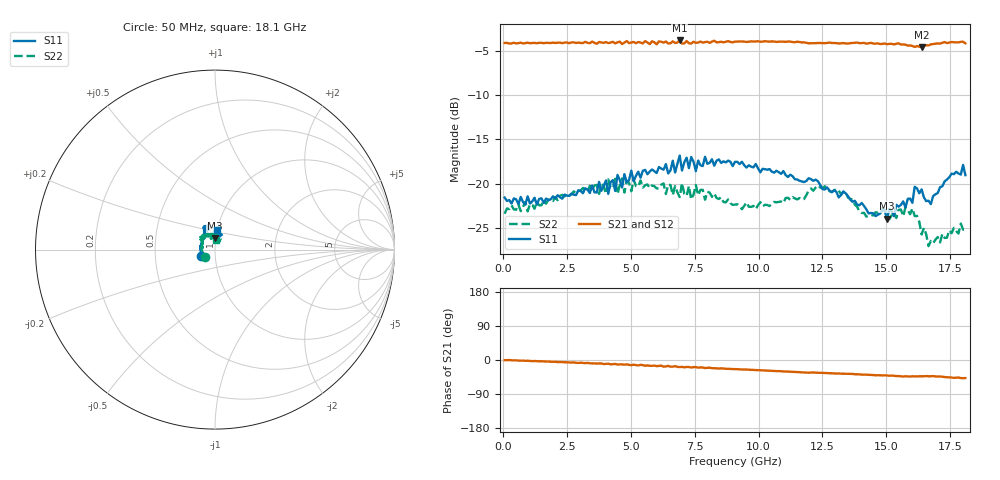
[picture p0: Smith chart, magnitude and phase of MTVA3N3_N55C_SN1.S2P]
! Network Analyzer HP8720D.06.14 Serial No. US36140669
! 27 Jun 2005  08:34:29
! Frequency  S11  S21  S12  S22
# HZ  S  DB R 50
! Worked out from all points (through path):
!   201 points, 50 MHz to 18.1 GHz, reference 50 ohm
!   highest |S21| = -3.81 dB at 6.909 GHz (marker M1); lowest = -4.6 dB at 16.39 GHz (marker M2)
!   group delay of S21, straight-line fit = 7.54 ps
!   lowest |S11| = -24.0 dB at 15.03 GHz (marker M3), VSWR 1.14, Z = 49.6 + j6.31 ohm
!   |S11| at or under -10 dB: start of sweep to end of sweep
!   |S22| runs from -27.1 to -19.4 dB; largest |S21 - S12| = 0.02
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5e7  -21.58 -155.5  -4.09 -0.5  -4.12 -0.1  -23.41 -142.0
3.1185e9  -21.09 137.7  -4.11 -7.8  -4.11 -8.0  -20.50 144.8
6.09675e9  -18.13 115.8  -3.91 -15.7  -3.90 -15.5  -20.54 123.5
6.45775e9  -18.86 118.1  -4.15 -15.4  -4.18 -16.4  -20.11 118.0
6.63825e9  -17.42 115.3  -3.90 -17.6  -4.03 -16.9  -21.31 117.9
6.7285e9  -18.75 117.8  -4.09 -16.2  -4.17 -17.4  -20.28 115.8
6.909e9  -16.83 114.8  -3.81 -18.5  -4.00 -17.9  -21.53 112.7
6.99925e9  -18.53 113.1  -4.15 -18.1  -4.11 -19.4  -19.95 113.7
7.36025e9  -16.99 104.8  -4.16 -19.9  -4.07 -18.7  -21.79 117.4
7.54075e9  -18.60 106.4  -4.07 -18.7  -3.88 -19.9  -20.17 116.3
7.90175e9  -16.97 111.5  -3.99 -21.3  -4.00 -20.3  -21.84 107.4
9.075e9  -17.54 115.9  -3.94 -23.9  -3.93 -24.0  -22.38 94.3
1.21435e10  -19.69 119.2  -4.11 -32.9  -4.09 -33.0  -20.82 93.6
1.50315e10  -23.96 89.9  -4.23 -40.8  -4.21 -41.5  -23.55 100.8
1.512175e10  -22.86 87.0  -4.19 -41.5  -4.12 -41.1  -24.03 98.1
1.602425e10  -22.18 76.8  -4.43 -43.0  -4.52 -44.4  -22.82 71.3
1.61145e10  -20.36 73.6  -4.54 -43.1  -4.35 -43.4  -23.70 69.8
1.638525e10  -20.66 65.8  -4.58 -43.0  -4.42 -42.6  -25.77 60.4
1.674625e10  -22.33 77.6  -4.25 -42.9  -4.35 -43.3  -26.50 67.6
1.75585e10  -18.88 86.7  -3.98 -46.1  -3.99 -46.5  -25.63 82.1
1.800975e10  -17.89 82.3  -3.95 -48.0  -3.95 -48.4  -25.22 88.4
1.81e10  -19.05 83.6  -4.13 -47.6  -4.16 -48.7  -25.19 84.6
